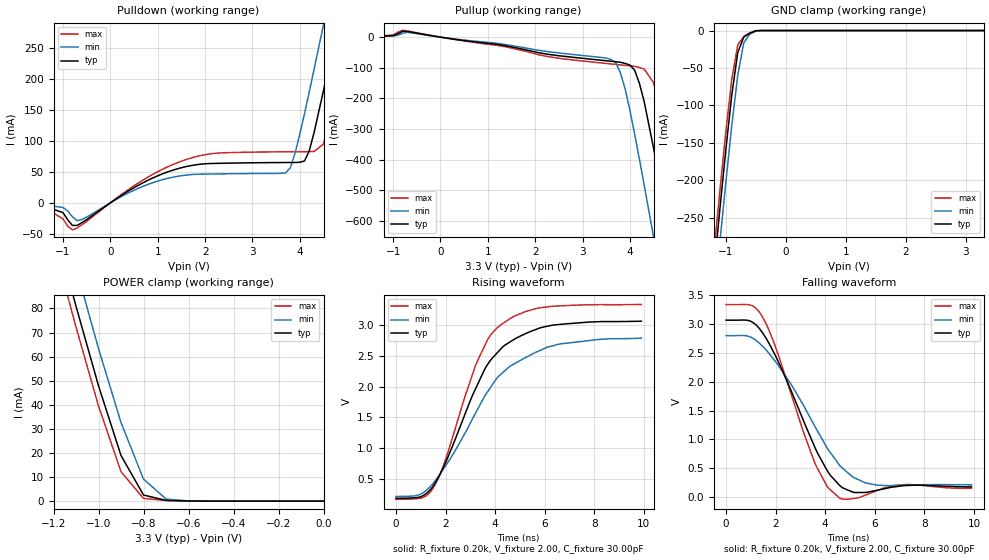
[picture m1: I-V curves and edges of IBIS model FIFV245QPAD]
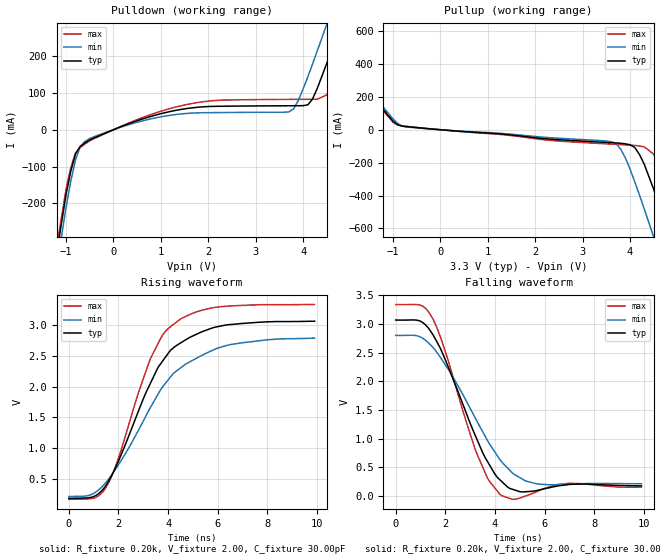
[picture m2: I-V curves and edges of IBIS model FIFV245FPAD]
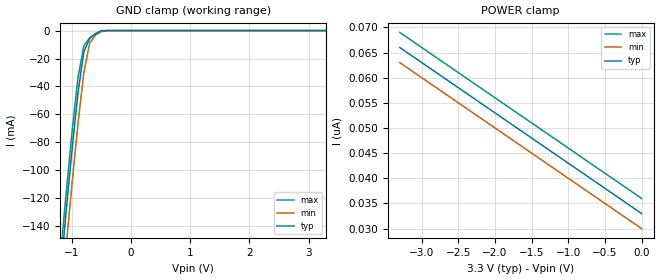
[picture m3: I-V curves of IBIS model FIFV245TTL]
| IBIS file i72v845.ibs created by s2ibis2 version 1.1
| North Carolina State University Electronics Research Laboratory  1995
[IBIS ver]   2.1
[File name]   i72v845.ibs
[File Rev]   1.0
[Date]   01/04/1999
[Source]   Integrated Device Technology, Inc.
[Notes]   1. Temperatures: typ=25C, min=70C, max=0C 2. Cemos8_3.3V
   process. 3. Ramp rates based on 50 ohm load.
[Copyright]   Copyright 1998, Integrated Device Technology, Inc.
|   Component idt72V845
[Component]   idt72V845
[Manufacturer]   Integrated Device Technology
[Package]
| variable   typ   min   max
R_pkg   0.75   0.60   0.90
L_pkg   8.10nH   8.30nH   9.90nH
C_pkg   0.53pF   0.46pF   0.60pF
[Pin]  signal_name   model_name   R_pin   L_pin   C_pin
1   VCC   POWER
2   PAFLA   FIFV245FPAD
3   RXILA   FIFV245TTL
4   FFLA   FIFV245FPAD
5   WXOLHFA   FIFV245FPAD
6   RXOLA   FIFV245FPAD
7   QA0   FIFV245QPAD
8   QA1   FIFV245QPAD
9   GND   GND
10   QA2   FIFV245QPAD
11   QA3   FIFV245QPAD
12   VCC   POWER
13   QA4   FIFV245QPAD
14   GND   GND
15   QA5   FIFV245QPAD
16   QA6   FIFV245QPAD
17   QA7   FIFV245QPAD
18   QA8   FIFV245QPAD
19   GND   GND
20   DB7   FIFV245TTL
21   DB6   FIFV245TTL
22   DB5   FIFV245TTL
23   DB4   FIFV245TTL
24   DB3   FIFV245TTL
25   DB2   FIFV245TTL
26   DB1   FIFV245TTL
27   DB0   FIFV245TTL
28   PAELB   FIFV245FPAD
29   FLBB   FIFV245TTL
30   WCLKB   FIFV245TTL
31   WENLB   FIFV245TTL
32   WXILB   FIFV245TTL
33   VCC   POWER
34   PAFLB   FIFV245FPAD
35   RXILB   FIFV245TTL
36   FFLB   FIFV245FPAD
37   WXOLHFB   FIFV245FPAD
38   RXOLB   FIFV245FPAD
39   QB0   FIFV245QPAD
40   QB1   FIFV245QPAD
41   GND   GND
42   QB2   FIFV245QPAD
43   QB3   FIFV245QPAD
44   VCC   POWER
45   QB4   FIFV245QPAD
46   GND   GND
47   QB5   FIFV245QPAD
48   QB6   FIFV245QPAD
49   QB7   FIFV245QPAD
50   QB8   FIFV245QPAD
51   GND   GND
52   QB9   FIFV245QPAD
53   QB10   FIFV245QPAD
54   VCC   POWER
55   QB11   FIFV245QPAD
56   QB12   FIFV245QPAD
57   GND   GND
58   QB13   FIFV245QPAD
59   QB14   FIFV245QPAD
60   VCC   POWER
61   QB15   FIFV245QPAD
62   GND   GND
63   QB16   FIFV245QPAD
64   QB17   FIFV245QPAD
65   EFLB   FIFV245FPAD
66   GND   GND
67   VCC   POWER
68   RSLB   FIFV245TTL
69   OELB   FIFV245TTL
70   LDLB   FIFV245TTL
71   RENLB   FIFV245TTL
72   RCLKB   FIFV245TTL
73   GND   GND
74   DB17   FIFV245TTL
75   DB16   FIFV245TTL
76   DB15   FIFV245TTL
77   DB14   FIFV245TTL
78   DB13   FIFV245TTL
79   DB12   FIFV245TTL
80   DB11   FIFV245TTL
81   DB10   FIFV245TTL
82   DB9   FIFV245TTL
83   DB8   FIFV245TTL
84   QA9   FIFV245QPAD
85   QA10   FIFV245QPAD
86   VCC   POWER
87   QA11   FIFV245QPAD
88   QA12   FIFV245QPAD
89   GND   GND
90   QA13   FIFV245QPAD
91   QA14   FIFV245QPAD
92   VCC   POWER
93   QA15   FIFV245QPAD
94   GND   GND
95   QA16   FIFV245QPAD
96   QA17   FIFV245QPAD
97   EFLA   FIFV245FPAD
98   GND   GND
99   VCC   POWER
100   RSLA   FIFV245TTL
101   OELA   FIFV245TTL
102   LDLA   FIFV245TTL
103   RENLA   FIFV245TTL
104   RCLKA   FIFV245TTL
105   GND   GND
106   DA17   FIFV245TTL
107   DA16   FIFV245TTL
108   DA15   FIFV245TTL
109   DA14   FIFV245TTL
110   DA13   FIFV245TTL
111   DA12   FIFV245TTL
112   DA11   FIFV245TTL
113   DA10   FIFV245TTL
114   DA9   FIFV245TTL
115   DA8   FIFV245TTL
116   DA7   FIFV245TTL
117   DA6   FIFV245TTL
118   DA5   FIFV245TTL
119   DA4   FIFV245TTL
120   DA3   FIFV245TTL
121   DA2   FIFV245TTL
122   DA1   FIFV245TTL
123   DA0   FIFV245TTL
124   PAELA   FIFV245FPAD
125   FLBA   FIFV245TTL
126   WCLKA   FIFV245TTL
127   WENLA   FIFV245TTL
128   WXILA   FIFV245TTL
| Models and submodels in the file (3): FIFV245QPAD (3-state), FIFV245FPAD (Output), FIFV245TTL (Input)
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| FIN  FIN   dummy_model
| QIN  QIN   dummy_model
| QOEL QOEL   dummy_model
|   Model FIFV245QPAD
[Model]   FIFV245QPAD
Model_type   3-state
Polarity   Non-Inverting
Enable   Active-Low
Vmeas =  1.500V
C_comp   3.00pF   NA   NA
[Temperature Range]   25.00   70.00   0.000
[Voltage Range]   3.30V   3.00V   3.60V
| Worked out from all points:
|   slope of the pulldown table from 0 to 0.495 V, typ, clamps not added: 20.4 ohm
|   slope of the pullup table from 0 to 0.495 V, typ, clamps not added: 44.7 ohm
|   GND clamp passes 1 mA (typ) near -0.52 V on its own axis
|   POWER clamp passes 1 mA (typ) near -0.73 V on its own axis
|   rising waveform, R_fixture 0.20k, V_fixture 2.00, C_fixture 30.00pF: 20-80 % time 1.95ns typ, 2.41ns min, 1.64ns max; typ from 0.181 V to 3.07 V
|   falling waveform, R_fixture 0.20k, V_fixture 2.00, C_fixture 30.00pF: 20-80 % time 1.76ns typ, 2.17ns min, 1.5ns max; typ from 3.07 V to 0.177 V
[Pulldown]
| voltage   I(typ)   I(min)   I(max)
-3.3V     -1mA       -1mA       0A
-1.5V     -2.7mA     -2.1mA     -3.3mA
-800mV    -36.55mA   -22.69mA   -43.77mA
1.5V      56.64mA    43.75mA    67.16mA
3.7V      65mA       48.37mA    82.35mA
3.9V      65.11mA    80.12mA    82.43mA
4.1V      67.6mA     144mA      82.48mA
4.5V      181mA      287mA      94.75mA
4.7V      253mA      361mA      155mA
4.9V      326mA      435mA      225mA
5.1V      400mA      510mA      298mA
6.6V      966mA      1.076A     862mA
[Pullup]
| voltage   I(typ)   I(min)   I(max)
-3.3V     300uA      300uA      300uA
-800mV    19.13mA    12.44mA    22.38mA
3.6V      -78.68mA   -72.88mA   -87.52mA
3.7V      -80.24mA   -82.94mA   -89.09mA
3.9V      -85.87mA   -170mA     -92.22mA
4.1V      -108mA     -317mA     -95.4mA
4.3V      -210mA     -482mA     -104mA
4.5V      -363mA     -653mA     -149mA
4.7V      -531mA     -826mA     -270mA
4.9V      -703mA     -1A        -430mA
5.1V      -878mA     -1.176A    -601mA
6.6V      -2.207A    -2.508A    -1.926A
[GND_clamp]
| voltage   I(typ)   I(min)   I(max)
-3.3V     -2.171A    -2.212A    -2.149A
-1.2V     -323mA     -367mA     -298mA
-1.1V     -240mA     -284mA     -216mA
-1V       -160mA     -204mA     -136mA
-900mV    -86.07mA   -127mA     -65.05mA
-800mV    -29.34mA   -59.59mA   -19.24mA
-700mV    -8.788mA   -16.49mA   -7.804mA
-600mV    -3.672mA   -4.887mA   -3.17mA
-500mV    -365uA     -944uA     -138uA
-400mV    -14.29nA   -611nA     -4.611nA
3.3V      33nA       33.88nA    33nA
[POWER_clamp]
| voltage   I(typ)   I(min)   I(max)
-3.3V     901mA      915mA      893mA
-1.2V     116mA      132mA      107mA
-1.1V     80.92mA    96.84mA    72.29mA
-1V       47.89mA    63.39mA    39.51mA
-900mV    18.95mA    32.6mA     12.21mA
-800mV    2.533mA    9.147mA    1.14mA
-700mV    314uA      878uA      268uA
-600mV    64.82uA    96.03uA    58.5uA
0V        33nA       30nA       36nA
[Ramp]
| variable   typ   min   max
dV/dt_r   1.03/1.09n   0.87/1.27n   1.19/0.99n
dV/dt_f   1.35/1.45n   1.13/1.85n   1.54/1.17n
R_load = 50.00
[Rising Waveform]
R_fixture = 0.20k
V_fixture = 2.00
C_fixture = 30.00pF
R_dut = 0.75
L_dut = 8.10nH
C_dut = 0.53pF
| time   V(typ)   V(min)   V(max)
0s        181mV      211mV      165mV
1ns       207mV      250mV      183mV
1.5ns     380mV      424mV      346mV
2ns       761mV      708mV      812mV
3.2ns     1.956V     1.561V     2.333V
3.7ns     2.364V     1.92V      2.767V
4.2ns     2.601V     2.19V      2.998V
5.2ns     2.859V     2.468V     3.22V
6.4ns     3.007V     2.675V     3.312V
9.9ns     3.067V     2.791V     3.339V
[Falling Waveform]
R_fixture = 0.20k
V_fixture = 2.00
C_fixture = 30.00pF
R_dut = 0.75
L_dut = 8.10nH
C_dut = 0.53pF
| time   V(typ)   V(min)   V(max)
0s        3.068V     2.8V       3.338V
1ns       3.048V     2.773V     3.327V
1.5ns     2.831V     2.606V     3.1V
2ns       2.445V     2.345V     2.598V
3.6ns     846mV      1.212V     571mV
4.1ns     445mV      835mV      168mV
4.6ns     195mV      542mV      -23.03mV
6.1ns     119mV      207mV      115mV
7.3ns     201mV      207mV      218mV
9.9ns     177mV      213mV      152mV
|   Model FIFV245FPAD
[Model]   FIFV245FPAD
Model_type   Output
Vmeas =  1.500V
C_comp   3.00pF   NA   NA
[Temperature Range]   25.00   70.00   0.000
[Voltage Range]   3.30V   3.00V   3.60V
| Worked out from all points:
|   slope of the pulldown table from 0 to 0.495 V, typ, clamps not added: 20.4 ohm
|   slope of the pullup table from 0 to 0.495 V, typ, clamps not added: 44.7 ohm
|   rising waveform, R_fixture 0.20k, V_fixture 2.00, C_fixture 30.00pF: 20-80 % time 1.94ns typ, 2.4ns min, 1.63ns max; typ from 0.181 V to 3.07 V
|   falling waveform, R_fixture 0.20k, V_fixture 2.00, C_fixture 30.00pF: 20-80 % time 1.62ns typ, 2.05ns min, 1.36ns max; typ from 3.07 V to 0.176 V
[Pulldown]
| voltage   I(typ)   I(min)   I(max)
-3.3V     -2.793A    -2.213A    -2.149A
-1.5V     -582mA     -626mA     -558mA
-1V       -176mA     -211mA     -162mA
-800mV    -65.89mA   -82.28mA   -63.01mA
-400mV    -21.63mA   -18.48mA   -23.86mA
1.6V      58.46mA    44.74mA    69.8mA
3.7V      65mA       48.37mA    82.35mA
4.1V      67.6mA     144mA      82.48mA
4.5V      181mA      287mA      94.75mA
4.7V      253mA      361mA      155mA
5.1V      400mA      510mA      298mA
6.6V      966mA      1.076A     862mA
[Pullup]
| voltage   I(typ)   I(min)   I(max)
-3.3V     901mA      915mA      893mA
-2.5V     598mA      613mA      590mA
-900mV    29.8mA     38.77mA    28.31mA
3.6V      -78.68mA   -72.88mA   -87.52mA
3.9V      -85.87mA   -170mA     -92.22mA
4.1V      -108mA     -317mA     -95.4mA
4.3V      -210mA     -482mA     -104mA
4.5V      -363mA     -653mA     -149mA
4.7V      -531mA     -826mA     -270mA
4.9V      -703mA     -1A        -430mA
5.1V      -878mA     -1.176A    -601mA
6.6V      -2.207A    -2.508A    -1.926A
[Ramp]
| variable   typ   min   max
dV/dt_r   1.03/1.07n   0.87/1.29n   1.19/0.96n
dV/dt_f   1.35/1.23n   1.13/1.60n   1.54/1.03n
R_load = 50.00
[Rising Waveform]
R_fixture = 0.20k
V_fixture = 2.00
C_fixture = 30.00pF
R_dut = 0.75
L_dut = 8.10nH
C_dut = 0.53pF
| time   V(typ)   V(min)   V(max)
0s        181mV      211mV      165mV
1ns       210mV      260mV      183mV
1.5ns     393mV      443mV      363mV
2ns       788mV      728mV      837mV
3.3ns     2.067V     1.67V      2.468V
3.8ns     2.43V      2.009V     2.856V
4.1ns     2.595V     2.161V     2.978V
5.1ns     2.846V     2.454V     3.213V
6.4ns     3.009V     2.676V     3.312V
9.9ns     3.067V     2.791V     3.339V
[Falling Waveform]
R_fixture = 0.20k
V_fixture = 2.00
C_fixture = 30.00pF
R_dut = 0.75
L_dut = 8.10nH
C_dut = 0.53pF
| time   V(typ)   V(min)   V(max)
0s        3.068V     2.8V       3.338V
1ns       3.047V     2.771V     3.327V
1.5ns     2.812V     2.59V      3.088V
3.2ns     1.059V     1.362V     814mV
3.7ns     598mV      964mV      309mV
4.2ns     280mV      631mV      25.41mV
5ns       74.15mV    319mV      -37.61mV
5.7ns     96.8mV     209mV      77.59mV
7ns       200mV      204mV      221mV
9.9ns     176mV      212mV      154mV
|   Model FIFV245TTL
[Model]   FIFV245TTL
Model_type   Input
Vinl =  0.000V
Vinh =  3.000V
Vmeas =  1.500V
C_comp   3.00pF   NA   NA
[Temperature Range]   25.00   70.00   0.000
[Voltage Range]   3.30V   3.00V   3.60V
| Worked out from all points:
|   GND clamp passes 1 mA (typ) near -0.54 V on its own axis
[GND_clamp]
| voltage   I(typ)   I(min)   I(max)
-3.3V     -1.215A    -1.238A    -1.203A
-1.2V     -177mA     -201mA     -164mA
-1.1V     -130mA     -155mA     -117mA
-1V       -85.9mA    -110mA     -73.09mA
-900mV    -45.15mA   -67.03mA   -34.14mA
-800mV    -15.42mA   -30.38mA   -11.05mA
-700mV    -5.554mA   -8.773mA   -5.066mA
-600mV    -2.384mA   -3.102mA   -2.034mA
-500mV    -209uA     -595uA     -61.81uA
-400mV    -8.386nA   -263nA     -4.26nA
3.3V      33nA       33nA       33nA
[POWER_clamp]
| voltage   I(typ)   I(min)   I(max)
-3.3V     66nA       63nA       69nA
-3.2V     65nA       62nA       68nA
-3V       63nA       60nA       66nA
0V        33nA       30nA       36nA
